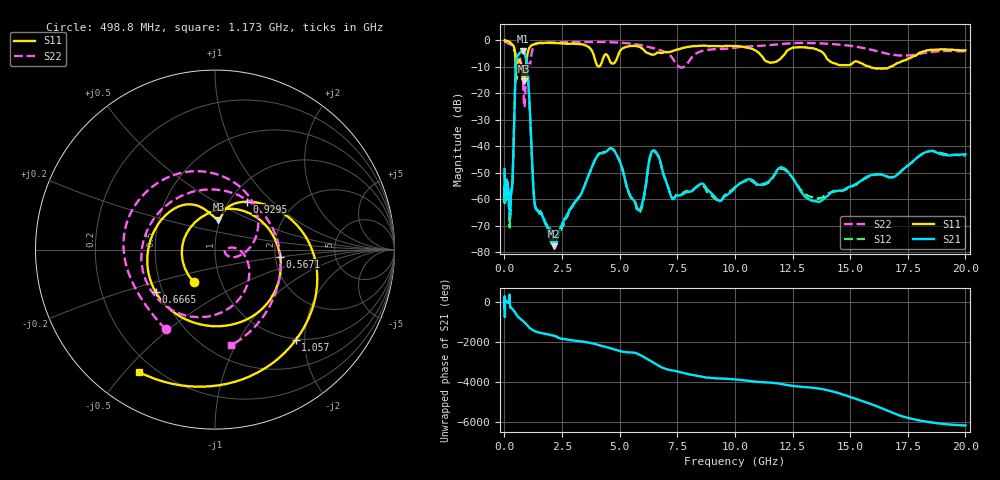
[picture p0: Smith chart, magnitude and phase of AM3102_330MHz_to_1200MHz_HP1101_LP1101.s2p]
! Date/Time: Tue, Sep 11, 2018 5:22 PM
! Network Analyzer: Agilent Technologies E8362B Rev: A.07.50.63
! Sweep from 0.010 to 20.000 GHz, 1601 Points, Sweep Type: LOG
! Power Supply: 4.949 V, 0.001 A
# Hz S DB R 50
!freq MagS11 AngS11 MagS21 AngS21 MagS12 AngS12 MagS22 AngS22
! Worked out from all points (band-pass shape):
!   1601 points, 10 MHz to 20 GHz, reference 50 ohm
!   highest |S21| = -4.00 dB at 798.4 MHz (marker M1); lowest = -77.8 dB at 2.165 GHz (marker M2)
!   |S21| within 3 dB of the highest: 520.2 MHz to 944.7 MHz (424.5 MHz wide, 58 % of centre)
!   lowest |S11| = -15.5 dB at 837.2 MHz (marker M3), VSWR 1.40, Z = 49.1 + j16.9 ohm
!   |S11| at or under -10 dB: 486.7 MHz to 552.3 MHz (65.66 MHz wide, 12.6 % of centre); 744.6 MHz to 927.8 MHz (183.2 MHz wide, 21.9 % of centre); 15.86 GHz to 16.74 GHz (883.5 MHz wide, 5.42 % of centre)
!   |S22| runs from -25.2 to -0.2 dB; largest |S21 - S12| = 0.0095
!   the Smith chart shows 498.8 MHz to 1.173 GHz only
!   S11 on the Smith chart (normalised r, x): 498.8 MHz: 0.74, -0.28; 567.1 MHz: 2.13, -0.19; 666.5 MHz: 0.46, -0.26; 929.5 MHz: 1.20, +0.71; 1.057 GHz: 0.97, -1.81; 1.173 GHz: 0.14, -0.55
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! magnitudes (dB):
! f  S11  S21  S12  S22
! 10 MHz  0.0  -48.7  -49.7  -0.2
! 35.55 MHz  -0.1  -60.0  -59.4  -0.5
! 126.4 MHz  -0.2  -54.3  -54.7  -1.0
! 238.9 MHz  -0.7  -65.2  -69.5  -1.4
! 352.7 MHz  -1.7  -53.4  -52.9  -2.5
! 447.2 MHz  -3.6  -21.6  -21.7  -4.1
! 498.8 MHz  -13.3  -9.0  -9.1  -5.7
! 567.1 MHz  -8.7  -5.9  -5.8  -5.9
! 666.5 MHz  -7.8  -4.8  -4.9  -6.7
! 798.4 MHz  -13.7  -4.0  -4.1  -14.3
! 837.2 MHz  -15.5  -4.1  -4.2  -21.7
! 929.5 MHz  -9.9  -6.2  -6.3  -14.1
! 1.057 GHz  -3.4  -18.4  -18.4  -8.8
! 1.173 GHz  -1.9  -40.2  -40.1  -5.3
! 1.59 GHz  -1.0  -65.3  -65.1  -0.9
! 2.165 GHz  -1.0  -77.8  -76.6  -0.7
! 4.5 GHz  -6.2  -41.4  -41.2  -0.6
! 5.652 GHz  -2.1  -60.9  -61.2  -1.4
! 6.518 GHz  -5.3  -41.7  -42.0  -3.0
! 7.41 GHz  -3.6  -59.0  -58.9  -8.3
! 13.48 GHz  -3.3  -60.8  -59.6  -1.1
! 20 GHz  -3.8  -43.1  -43.6  -4.2
